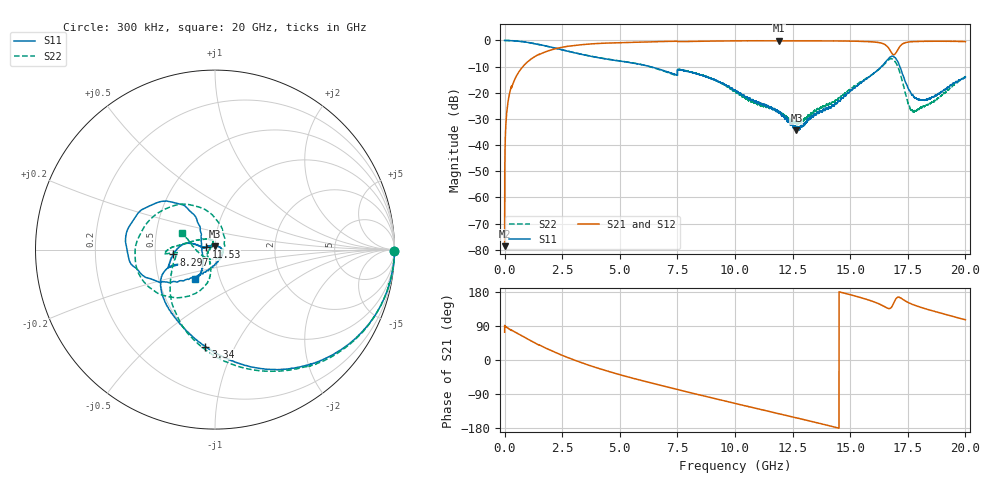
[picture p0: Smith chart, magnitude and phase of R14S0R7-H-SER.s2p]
!{R14S0R7}
!Johanson Technology Inc.
!www.johansontechnology.com
!Test Board Conditions:
!Substrate Type  RO4350B
!Substrate Thickness  20 mil
!Substrate Dk  3.66
!TL Type: GCPW
!TL Trace Width  36 mil
!TL Gap  12 mil
!Electrode orientation  Horizontal
!DUT TOPOLOGY	SERIES
!Mounting Pad LxW  26x36 mil
! Created Wed Nov 25 17:33:21 2020
! 2 Port Network Data from SP1.SP block
! freq  magS11  angS11  magS21  angS21  magS12  angS12  magS22  angS22
# khz S ma R 50
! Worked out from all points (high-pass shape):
!   20001 points, 300 kHz to 20 GHz, reference 50 ohm
!   highest |S21| = -0.10 dB at 11.92 GHz (marker M1); lowest = -78.6 dB at 300 kHz (marker M2)
!   |S21| within 3 dB of the highest: 2.234 GHz to 16.68 GHz (14.45 GHz wide, 153 % of centre); 17.1 GHz to end of sweep
!   lowest |S11| = -34.3 dB at 12.67 GHz (marker M3), VSWR 1.04, Z = 49.9 + j1.92 ohm
!   |S11| at or under -10 dB: 6.324759 GHz to 6.32568 GHz (921.4 kHz wide, 0.0146 % of centre); 6.33 GHz to 16.36 GHz (10.03 GHz wide, 88.4 % of centre); 17.15 GHz to end of sweep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
!   |S22| runs from -32.1 to 0.0 dB; largest |S21 - S12| = 0.013
!   S11 on the Smith chart (normalised r, x): 300 kHz: open; 3.34 GHz: 0.50, -0.77; 8.297 GHz: 0.62, -0.04; 11.53 GHz: 0.90, +0.03; 20 GHz: 0.76, -0.26
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300  0.9995 -0.3  0.0001174 73.3  0.0001046 65.0  0.9991 -0.3
101300  0.9982 -3.9  0.04603 85.9  0.04623 85.9  0.9989 -3.9
132300  0.9979 -5.0  0.06003 84.7  0.06032 84.7  0.9979 -5.1
507300  0.9765 -17.7  0.2069 71.8  0.2073 72.0  0.9764 -17.8
1684300  0.8038 -54.7  0.5848 34.4  0.5853 34.3  0.8032 -55.9
3334300  0.5436 -95.6  0.829 -6.9  0.8303 -7.0  0.5458 -98.0
3340300  0.5426 -95.7  0.8297 -7.1  0.8304 -7.1  0.5451 -98.2
6667300  0.2868 -158.4  0.9491 -65.2  0.9498 -65.1  0.2821 -150.4
8297300  0.2332 -173.3  0.9616 -89.8  0.9621 -89.6  0.2354 176.6
1.00003e7  0.1126 165.3  0.9826 -114.5  0.9817 -114.5  0.1055 148.6
1.15293e7  0.05315 163.9  0.9858 -136.4  0.9864 -136.4  0.05074 103.5
1.19203e7  0.04104 152.0  0.9884 -142.1  0.9858 -142.0  0.04278 105.3
1.26683e7  0.01926 93.2  0.9838 -152.7  0.9827 -152.7  0.02672 145.1
1.33343e7  0.03524 11.5  0.9831 -162.3  0.9856 -162.3  0.04063 -160.9
1.55863e7  0.1675 -122.4  0.9577 162.3  0.9566 162.3  0.1766 -101.9
1.66673e7  0.45 -166.4  0.7174 135.8  0.7075 136.2  0.4255 -151.4
1.68533e7  0.5012 168.4  0.5398 145.7  0.5335 146.4  0.4357 173.5
1.70653e7  0.3951 137.0  0.6637 165.6  0.6621 166.4  0.3174 127.2
1.73113e7  0.2061 120.8  0.8777 159.0  0.8774 159.4  0.1378 76.4
1.77233e7  0.08955 148.1  0.9486 146.3  0.9508 146.1  0.04387 -22.9
1.84183e7  0.07782 -152.5  0.9658 132.5  0.962 132.6  0.06175 -121.3
2e7  0.1968 -124.2  0.9515 106.0  0.9444 106.0  0.2047 152.8
